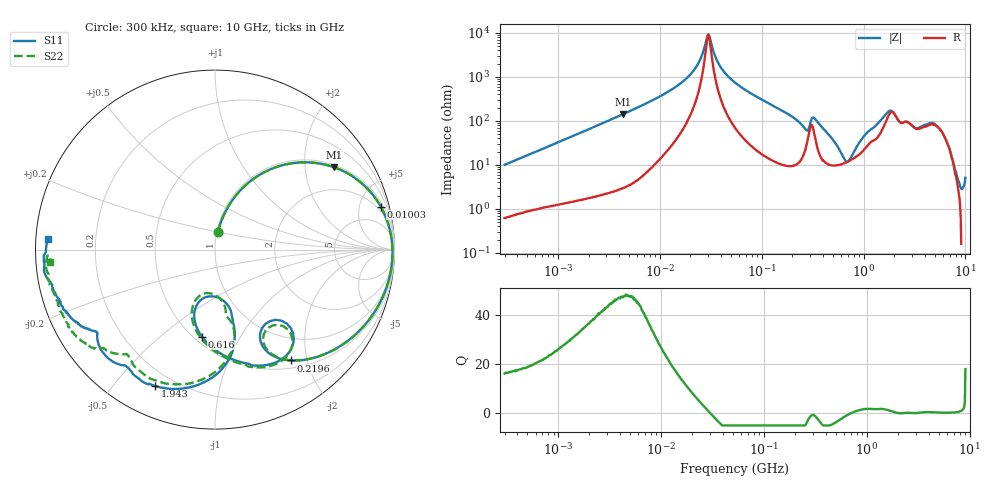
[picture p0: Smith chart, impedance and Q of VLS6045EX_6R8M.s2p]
! S-Parameter Data Generated by TDK Corporation
! Copyright(C) 2019 TDK Corporation.
! All Rights Reserved.
! TDK P/N: VLS6045EX-6R8M (Inductor)
! Property: L=6.8uH at 100kHz
! Size(LxWxT): 6x6x4.5mm
! Model Type: s2p (Touchstone File Format Version 1.0)
! Frequency: DC=Yes Start=0.3MHz Stop=10000MHz 802points Log-sweep
! Model Generated on May 10, 2019
! Port Assignments:
!  1 ---@@@--- 2
! Applicable Conditions:
!  Temperature = 25 degC
!  DC Bias Current = 0 A
!  Small Signal Operation
! Terms and conditions regarding TDK Simulation Models
! (1)This simulation model is being provided solely for informational purposes. Please refer to the specifications of the products in terms of detailed characteristics of such products.
! (2)In no event shall TDK Corporation of any of its subsidiaries be liable for any loss or damage arising, directly or indirectly,
!  From any information contained in this simulation model, including, but not limited to loss or damages arising from any inaccuracies, omissions or errors in connection with such information.
! (3)Any and all copyrights on this simulation model are owned by TDK Corporation.
!  Duplication or redistribution of this simulation model without prior written permission from TDK Corporation is prohibited.
! (4)This simulation model is subject to any modification or change without any prior notice.
! (5)Neither TDK Corporation nor any of its subsidiaries shall make any warranty, express or implied,
!  Including but not limited to the correctness, implied warranties of merchantability and fitness for a particular purpose with respect to this simulation models.
! (6)The use of this simulation model shall be deemed to have consented to the terms and conditions hereof.
# Hz S MA R 50
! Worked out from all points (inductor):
!   801 points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, 300 kHz to 10 GHz, reference 50 ohm
!   read as one part in series: L = 5.27 uH near 318.3 kHz
!   highest Q = 47.8 at 4.363 MHz (marker M1), where L = 5.16 uH
!   self-resonance near 29.88 MHz
!   S11 on the Smith chart (normalised r, x): 300 kHz: 1.01, +0.20; 10.03 MHz: 1.42, +7.57; 219.6 MHz: 0.62, -1.73; 616 MHz: 0.55, -0.70; 1.943 GHz: 0.13, -0.65; 10 GHz: 0.04, +0.03
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300000  0.09802 80.8  0.989 -5.8  0.9891 -5.8  0.09794 80.5
1713600  0.4754 59.8  0.8659 -28.5  0.8662 -28.5  0.4753 59.8
4363314  0.8081 34.5  0.5723 -54.3  0.5724 -54.3  0.8082 34.5
9671944  0.9507 15.3  0.2774 -72.7  0.2774 -72.7  0.9509 15.3
1.002822e7  0.9539 14.6  0.2661 -73.3  0.2661 -73.3  0.954 14.6
2.126252e7  0.9869 2.4  0.07348 -79.5  0.07349 -79.5  0.987 2.3
2.987769e7  0.9891 -2.5  0.01079 -7.5  0.01079 -7.4  0.9892 -2.5
3.904515e7  0.9872 -6.5  0.05621 72.0  0.05621 72.0  0.9873 -6.5
5.477226e7  0.979 -12.2  0.1315 72.4  0.1315 72.4  0.9791 -12.2
1.177683e8  0.9167 -30.7  0.3531 56.3  0.3531 56.3  0.9171 -30.6
2.195581e8  0.7481 -55.7  0.6018 29.7  0.6018 29.7  0.7503 -55.3
2.725454e8  0.5546 -63.1  0.6691 9.4  0.6691 9.4  0.5701 -61.9
3.126428e8  0.6387 -47.0  0.465 5.2  0.4651 5.2  0.6595 -49.2
3.7738e8  0.6944 -68.6  0.621 12.1  0.6211 12.1  0.6977 -70.2
6.15965e8  0.4898 -98.6  0.7727 -20.3  0.7728 -20.3  0.4879 -100.3
1.054047e9  0.2704 -85.4  0.6974 -72.0  0.6977 -72.0  0.2763 -83.9
1.403063e9  0.5492 -79.0  0.4742 -109.9  0.4746 -109.9  0.5292 -78.6
1.767019e9  0.7953 -103.3  0.1919 -122.1  0.1925 -122.0  0.7791 -105.5
1.942751e9  0.8304 -113.6  0.1539 -106.2  0.1549 -106.2  0.8041 -116.4
3.387826e9  0.8027 -144.8  0.1467 -123.4  0.1451 -124.0  0.8316 -138.7
5.284132e9  0.898 -157.7  0.05851 -142.7  0.05777 -141.9  0.9176 -152.8
1e10  0.9321 176.4  0.04217 -158.0  0.04273 -158.3  0.9238 -175.6
